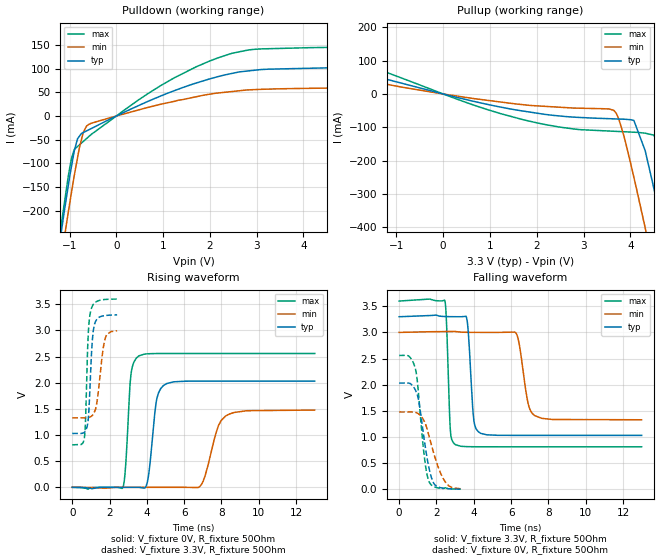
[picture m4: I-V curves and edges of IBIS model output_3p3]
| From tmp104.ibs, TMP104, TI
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|   output_3p3 Model
[Model]   output_3p3
Model_type   Output
Polarity   Non-Inverting
Vmeas = 1.65
Vref = 1.65
Cref = 2pF
Rref = 50
|   typ   min   max
|   (nom PVT)   (fast PVT)   (slow PVT)
|C_comp from frequency sweep method (F=0.001MHz)
|C_comp   2.613e-12   2.536e-12   2.698e-12
|ON state : BUFFER OUTPUT TURNED HIGH
|C_comp   2.613e-12   2.536e-12   2.698e-12
|OFF state: BUFFER OUTPUT TURNED LOW
|C_comp   1.770e-12   1.715e-12   1.834e-12
|C_comp from LC tank measurement(L=1nH)
|Resonant Frequency(Hz)   4.810e+09   5.130e+09   4.510e+09
C_comp   1.096e-12   9.635e-13   1.247e-12
|ON state : BUFFER OUTPUT TURNED HIGH
|Resonant Frequency(Hz)   4.810e+09   5.130e+09   4.510e+09
|C_comp   1.096e-12   9.635e-13   1.247e-12
|OFF state: BUFFER OUTPUT TURNED LOW
|Resonant Frequency(Hz)   5.770e+09   5.850e+09   5.520e+09
|C_comp   7.616e-13   7.409e-13   8.321e-13
| Where nom  PVT is Nominal Process, 3.3V, 25C
|   Fast PVT is Strong Process,  3.6V, -40C
|   Slow PVT is Weak Process,   3V, 125C
[Voltage Range]   3.3   3   3.6
|Ambient Temperature   25   125   -40
|Junction Temperature
[Temperature Range]   25   125   -40
[Pullup Reference]   3.3   3   3.6
[Pulldown Reference]   0   0   0
[Power Clamp Reference]   3.3   3   3.6
[GND Clamp Reference]   0   0   0
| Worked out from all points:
|   slope of the pulldown table from 0 to 0.495 V, typ, clamps not added: 21.7 ohm
|   slope of the pullup table from 0 to 0.495 V, typ, clamps not added: 29.1 ohm
|   falling waveform, V_fixture 3.3V, R_fixture 50Ohm: 20-80 % time 224ps typ, 412ps min, 156ps max; typ from 3.3 V to 1.03 V
|   rising waveform, V_fixture 0V, R_fixture 50Ohm: 20-80 % time 348ps typ, 662ps min, 237ps max; typ from 0 V to 2.03 V
|   rising waveform, V_fixture 3.3V, R_fixture 50Ohm: 20-80 % time 193ps typ, 323ps min, 156ps max; typ from 1.03 V to 3.3 V
|   falling waveform, V_fixture 0V, R_fixture 50Ohm: 20-80 % time 517ps typ, 755ps min, 410ps max; typ from 2.03 V to 0.002 V
[Pulldown]
|   Voltage   I(typ)   I(min)   I(max)
-3.3V     -1.758A    -1.778A    -1.774A
-1.325V   -346.6mA   -398.9mA   -329.3mA
-1.158V   -232.2mA   -287.2mA   -216.2mA
-1.122V   -207.5mA   -263.8mA   -191.8mA
-1.026V   -146.7mA   -202.7mA   -126.7mA
-896.4mV  -72.86mA   -124.3mA   -70.25mA
-636mV    -31.43mA   -21.3mA    -47.51mA
1.706V    69.48mA    40.58mA    103.7mA
2.83V     95.12mA    55.06mA    139.3mA
5.004V    102.8mA    61.36mA    145.2mA
5.803V    115mA      88.37mA    148.9mA
6.6V      147.4mA    115.3mA    187.5mA
[Pullup]
|   Voltage   I(typ)   I(min)   I(max)
-3.3V     146.7mA    105.8mA    198.5mA
-1.528V   56.01mA    38.61mA    81.56mA
939.6mV   -31.15mA   -19.03mA   -46.73mA
3.645V    -74.77mA   -49.22mA   -112mA
3.855V    -75.81mA   -122.6mA   -113.4mA
4.075V    -79.47mA   -250.5mA   -114.9mA
4.314V    -169.3mA   -400.1mA   -117.7mA
4.511V    -289.2mA   -527.9mA   -125.8mA
4.684V    -401.7mA   -646.1mA   -205.1mA
4.896V    -541.5mA   -791.4mA   -338.7mA
5.148V    -713mA     -967.9mA   -506.2mA
6.6V      -1.758A    -1.99A     -1.558A
[Ramp]
R_load = 50
|   typ   min   max
dV/dt_r   1.21832/3.46249e-10   0.886361/6.56272e-10   1.53548/2.36036e-10
dV/dt_f   1.36208/2.22316e-10   1.00283/4.09691e-10   1.67293/1.55695e-10
[Falling Waveform]
V_fixture = 3.3V
V_fixture_min = 3V
V_fixture_max = 3.6V
R_fixture = 50Ohm
|   Time   V(typ)   V(min)   V(max)
0s        3.3V       3V         3.6V
2.448ns   3.304V     3.017V     3.608V
2.744ns   3.301V     3.018V     1.136V
3.012ns   3.301V     3.018V     853.7mV
3.612ns   3.285V     3.003V     814.8mV
4ns       1.332V     3.001V     812.7mV
4.368ns   1.07V      3V         812.1mV
6.256ns   1.03V      2.991V     811.8mV
7.272ns   1.03V      1.407V     811.8mV
13ns      1.03V      1.329V     811.8mV
[Rising Waveform]
V_fixture = 0V
V_fixture_min = 0V
V_fixture_max = 0V
R_fixture = 50Ohm
|   Time   V(typ)   V(min)   V(max)
0s        412.2pV    1.087nV    371pV
2.712ns   -37.96uV   -131.9uV   -4.298mV
3.144ns   -14.09uV   -76.44uV   2.15V
3.588ns   -462uV     -31.06uV   2.515V
4.016ns   84.95mV    -13.91uV   2.552V
4.532ns   1.691V     -5.614uV   2.558V
5.064ns   1.984V     -2.45uV    2.559V
6.928ns   2.03V      55.59mV    2.559V
8.224ns   2.03V      1.364V     2.559V
13ns      2.031V     1.477V     2.559V
[Rising Waveform]
V_fixture = 3.3V
V_fixture_min = 3V
V_fixture_max = 3.6V
R_fixture = 50Ohm
|   Time   V(typ)   V(min)   V(max)
0s        1.03V      1.329V     811.8mV
648ps     1.051V     1.328V     940.2mV
716ps     1.08V      1.328V     1.333V
812ps     1.19V      1.33V      2.532V
860ps     1.32V      1.333V     2.952V
1.028ns   2.535V     1.36V      3.423V
1.112ns   2.949V     1.391V     3.489V
1.208ns   3.135V     1.458V     3.529V
1.772ns   3.284V     2.854V     3.592V
2.404ns   3.297V     2.993V     3.599V
[Falling Waveform]
V_fixture = 0V
V_fixture_min = 0V
V_fixture_max = 0V
R_fixture = 50Ohm
|   Time   V(typ)   V(min)   V(max)
0s        2.031V     1.477V     2.559V
528ps     2.03V      1.477V     2.543V
872ps     1.897V     1.47V      2.303V
948ps     1.831V     1.46V      2.148V
1.064ns   1.662V     1.434V     1.716V
1.36ns    909.9mV    1.292V     592mV
1.616ns   379.3mV    998.4mV    134.7mV
1.912ns   84.32mV    618.5mV    41.92mV
2.372ns   18.95mV    197.3mV    14.93mV
3.3ns     1.625mV    9.416mV    909.8uV
